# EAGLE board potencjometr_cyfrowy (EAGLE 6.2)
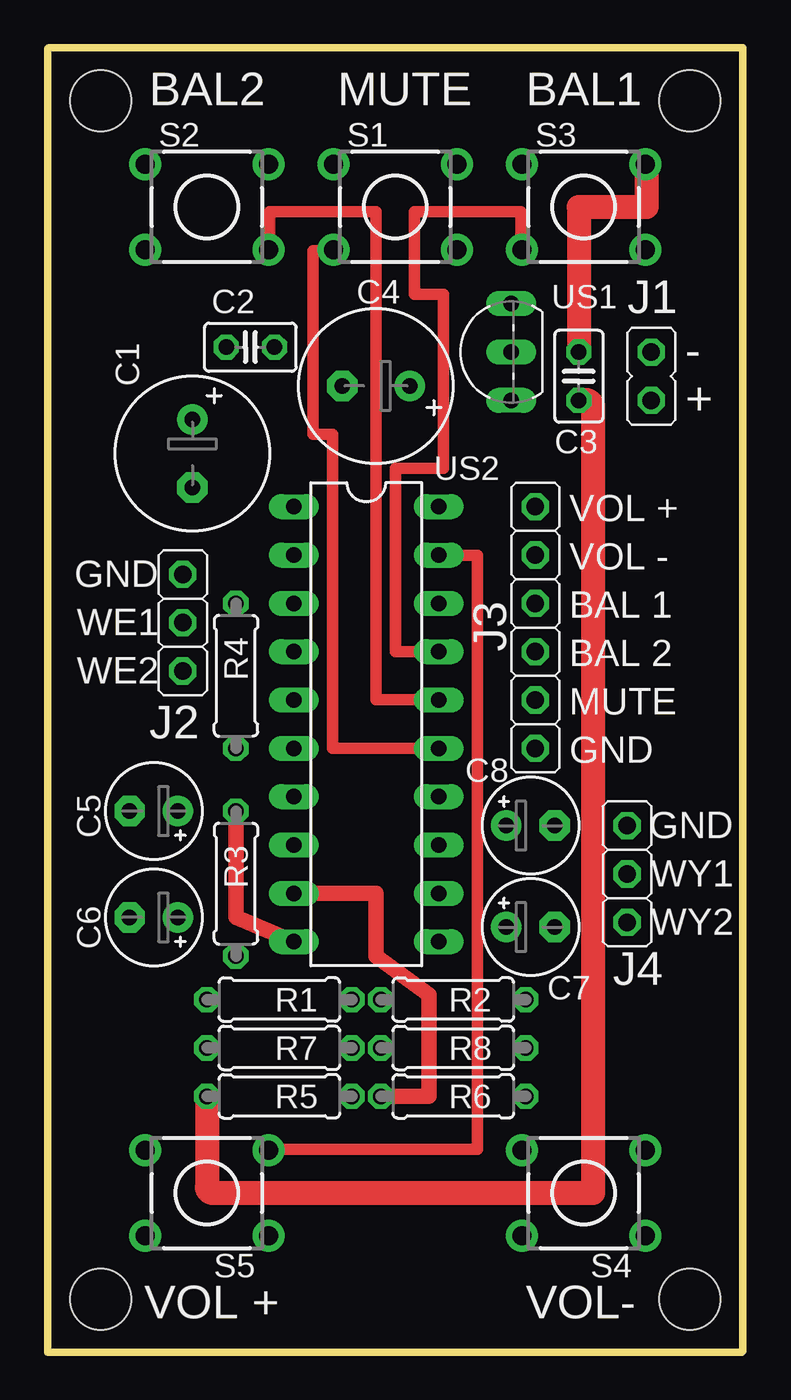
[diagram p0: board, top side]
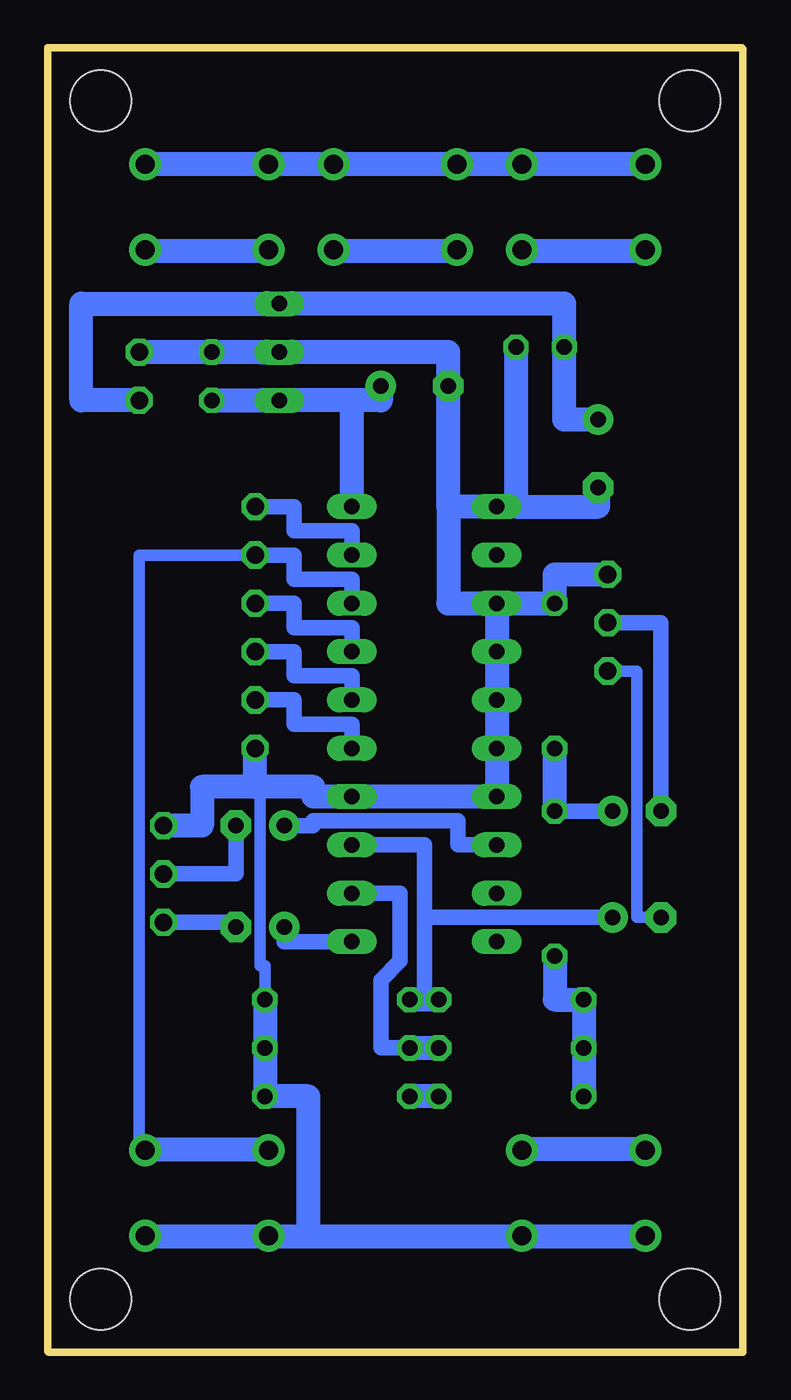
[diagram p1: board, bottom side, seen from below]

Size 36.58 x 68.58 mm. Coordinates in mm from the lower left corner, seen from the top.
Outline: 36.58,0.06 36.58,68.58 0.06,68.58
Outline: 36.51,0 0,0 0,68.52
Copper layers (1*16): Top 0.035mm / dielectric 1.5mm / Bottom 0.035mm
Design rules: minimum track width 10mil, minimum drill 24mil, track to track 8mil, track to pad 8mil, pad to pad 8mil, via to via 8mil, smd to smd 8mil, copper to edge 40mil, drill to drill 8mil, minimum pad ring 10mil, minimum via ring 8mil, stop-mask expansion 4mil, vias tented up to drill 0mil, thermal gap 10mil
Holes 3.2 mm at 2.79,65.79 33.78,65.79 2.79,2.79 33.78,2.79

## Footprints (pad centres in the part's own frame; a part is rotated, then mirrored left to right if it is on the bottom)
E3,5-8 = drill 0.813 pad 1.6: + -1.778,0 | drill 0.813 pad 1.6 octagon: - 1.778,0
C025-025X050 = drill 0.813 octagon: 1 -1.27,0; 2 1.27,0
E2,5-5 = drill 0.813 pad 1.6: + -1.27,0 | drill 0.813 pad 1.6 octagon: - 1.27,0
JUMPER_JP1 = drill 0.914 pad 1.422 octagon: 1 0,-1.27; 2 0,1.27
0207/7 = drill 0.813 octagon: 1 -3.81,0; 2 3.81,0
TL1105 = drill 1 pad 1.676: 1 -2.25,3.25; 2 2.25,3.25; 3 -2.25,-3.25; 4 2.25,-3.25
TO92- = drill 0.813 long: 1 2.54,0; 2 0,0; 3 -2.54,0
DIL20 = drill 0.813 long: 1 -11.43,-3.81; 2 -8.89,-3.81; 3 -6.35,-3.81; 4 -3.81,-3.81; 5 -1.27,-3.81; 6 1.27,-3.81; 7 3.81,-3.81; 8 6.35,-3.81; 9 8.89,-3.81; 10 11.43,-3.81; 11 11.43,3.81; 12 8.89,3.81; 13 6.35,3.81; 14 3.81,3.81; 15 1.27,3.81; 16 -1.27,3.81; 17 -3.81,3.81; 18 -6.35,3.81; 19 -8.89,3.81; 20 -11.43,3.81

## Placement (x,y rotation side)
C1  [E3,5-8]  7.62,47.24 270 top
C2  [C025-025X050]  10.67,52.83 180 top
C3  [C025-025X050]  27.94,51.31 270 top
C4  [E3,5-8]  17.27,50.8 180 top
C5  [E2,5-5]  5.59,28.45 180 top
C6  [E2,5-5]  5.59,22.86 180 top
C7  [E2,5-5]  25.4,22.35 0 top
C8  [E2,5-5]  25.4,27.69 0 top
E$16  [JUMPER_JP1]  7.11,39.62 0 top
E$17  [JUMPER_JP1]  7.11,37.08 0 top
E$20  [JUMPER_JP1]  30.48,23.88 0 top
E$21  [JUMPER_JP1]  30.48,26.42 0 top
E$22  [JUMPER_JP1]  25.65,33.02 0 top
E$23  [JUMPER_JP1]  25.65,35.56 0 top
E$24  [JUMPER_JP1]  25.65,38.1 0 top
E$25  [JUMPER_JP1]  25.65,40.64 0 top
E$26  [JUMPER_JP1]  25.65,43.18 0 top
E$32  [JUMPER_JP1]  31.75,51.31 0 top
R1  [0207/7]  12.19,18.54 180 top
R2  [0207/7]  21.34,18.54 180 top
R3  [0207/7]  9.91,24.64 270 top
R4  [0207/7]  9.91,35.56 270 top
R5  [0207/7]  12.19,13.46 180 top
R6  [0207/7]  21.34,13.46 180 top
R7  [0207/7]  12.19,16 180 top
R8  [0207/7]  21.34,16 180 top
S1  [TL1105]  18.29,60.2 270 top
S2  [TL1105]  8.38,60.2 270 top
S3  [TL1105]  28.19,60.2 270 top
S4  [TL1105]  28.19,8.38 90 top
S5  [TL1105]  8.38,8.38 90 top
US1  [TO92-]  24.38,52.58 90 top
US2  [DIL20]  16.76,33.02 270 top

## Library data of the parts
C1-C8 R1-R8 = rcl
E$16 E$17 E$20-E$26 E$32 = hybrid
S1-S5 = switch
US1 = transistor-npn
US2 = 40xx

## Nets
S$1: E$22.2 US2.15
S$3: C3.2 C4.+ R1.2 R3.2 R5.2 US2.20
S$4: C6.+ R1.1 R2.2 US2.13
S$6: R7.1 R8.2 US2.12
S$7: R5.1 R6.2 US2.9
S$8: C5.- E$16.1
S$9: C6.- E$17.1
S$10: C1.- C2.1 C3.1 E$16.2 E$21.2 E$22.1 E$32.2 R2.1 R4.1 R6.1 US2.1 US2.3 US2.7 US2.14
S$11: C7.+ US2.11
S$12: C8.+ US2.8
S$13: C7.- E$20.1
S$14: C8.- E$20.2
S$16: E$23.2 US2.16
S$17: E$24.2 US2.17
S$18: C1.+ C2.2 E$32.1
S$19: C5.+ R3.1 R4.2 US2.10
S$25: E$25.2 US2.18
S$26: E$26.2 US2.19

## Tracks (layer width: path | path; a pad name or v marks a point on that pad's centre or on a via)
S$1
  Top 0.61: US2.15 14.99,31.75 14.99,48.26 13.97,48.26 13.97,57.91 14.99,57.91
  Bottom 0.813: E$22.2 23.62,34.29 23.62,33.02 20.57,33.02 US2.15
S$3
  Top 1.27: R5.2 8.38,8.7 arc90 8.7,8.38 28.7,8.38 28.7,49.72 arc90 28.13,50.04 C3.2
  Bottom 1.27: R3.2 9.91,18.54 R1.2 R5.2 | C3.2 25.4,50.04 | 25.4,50.04 24.89,50.04 | C4.+ 19.05,50.04 20.57,50.04 | 20.57,50.04 25.4,50.04 | US2.20 20.57,50.04
S$4
  Bottom 0.813: 16.76,18.54 16.76,22.86 | 16.76,22.86 16.76,26.67 US2.13 | C6.+ 16.76,22.86
  Bottom 1.27: R1.1 16.76,18.54 R2.2
S$6
  Bottom 0.813: R8.2 19.05,16 19.05,19.56 18.03,20.57 18.03,24.13 US2.12
  Bottom 1.27: R8.2 R7.1
S$7
  Top 0.813: US2.9 17.27,24.13 17.27,20.83 20.07,18.8 20.07,13.46 R6.2
  Bottom 1.27: R5.1 R6.2
S$8
  Bottom 0.813: C5.- 4.32,38.35 E$16.1 7.11,38.1
S$9
  Bottom 0.61: C6.- 5.59,22.86 5.59,35.81 E$17.1
S$10
  Top 1.27: 31.5,62.48 31.5,60.2 27.94,60.2 C3.1
  Bottom 0.61: 25.4,18.54 R2.1 25.15,20.32 25.4,20.32 25.4,29.72
  Bottom 1.27: R2.1 R6.1 22.86,13.46 22.86,6.1 | E$21.2 28.45,27.69 28.45,29.72 25.65,29.72 | 25.65,29.72 E$22.1 | 25.65,29.72 25.4,29.72 22.61,29.72 22.61,29.21 US2.14 US2.7 US2.3 | 25.4,52.58 C3.1 E$32.2 | 25.4,52.58 24.89,52.58 | 25.4,52.58 15.49,52.58 15.49,44.45 | 15.49,44.45 US2.1 11.94,44.45 | 15.49,44.45 15.49,39.37 US2.3 | US2.3 R4.1 9.91,40.89 E$16.2 | C1.- 7.62,44.45 11.94,44.45 | C2.1 11.94,44.45
S$11
  Bottom 0.813: C7.+ 24.13,21.59 US2.11
S$12
  Bottom 0.813: US2.8 14.99,26.67 14.99,27.94 22.61,27.94 22.61,27.69 C8.+
S$13
  Bottom 0.813: C7.- 26.67,22.61 E$20.1
S$14
  Bottom 0.813: C8.- 26.67,25.15 E$20.2
S$15
  Bottom 1.27: 5.08,10.67 11.68,10.67
S$16
  Top 0.61: US2.16 17.27,34.29 17.27,59.94 11.68,59.94 11.68,57.91
  Bottom 0.813: E$23.2 23.62,36.83 23.62,35.56 20.57,35.56 US2.16
S$17
  Top 0.61: 18.29,40.13 18.29,46.48 20.83,46.48 20.83,55.63 19.3,55.63 19.3,59.94 24.89,59.94 24.89,57.91 | 18.29,40.13 18.29,39.37 | 18.29,40.13 18.29,36.83 US2.17
  Bottom 0.813: E$24.2 23.62,39.37 23.62,38.1 20.57,38.1 US2.17
S$18
  Bottom 1.27: E$32.1 34.8,50.04 34.8,55.12 23.62,55.12 | C1.+ 9.4,49.02 C2.2 9.4,55.12 23.62,55.12 | 23.62,55.12 24.89,55.12
S$19
  Top 0.813: US2.10 9.91,22.86 R3.1
  Bottom 0.813: C5.+ R3.1
  Bottom 1.27: R3.1 R4.2
S$20
  Bottom 1.27: 31.5,62.48 5.08,62.48
S$21
  Bottom 1.27: 31.5,57.91 24.89,57.91
S$22
  Bottom 1.27: 21.59,57.91 14.99,57.91
S$23
  Bottom 1.27: 11.68,57.91 5.08,57.91
S$24
  Bottom 1.27: 31.5,6.1 5.08,6.1
S$25
  Bottom 0.61: 31.5,10.67 31.75,10.67 31.75,41.91 E$25.2
  Bottom 0.813: E$25.2 23.62,41.91 23.62,40.64 20.57,40.64 US2.18
  Bottom 1.27: 31.5,10.67 24.89,10.67
S$26
  Top 0.61: US2.19 22.61,41.91 22.61,10.67 11.68,10.67
  Bottom 0.813: E$26.2 23.62,44.45 23.62,43.18 20.57,43.18 US2.19

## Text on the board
tNames: BAL2 | MUTE | BAL1 | J1 | - | + | VOL + | GND | VOL - | WE1 | BAL 1 | J3 | WE2 | BAL 2 | MUTE | J2 | GND | GND | WY1 | WY2 | J4 | VOL + | VOL-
